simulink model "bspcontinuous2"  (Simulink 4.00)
settings: Solver=ode45  StartTime=0.0  StopTime=25  FixedStep=0.01  RelTol=1e-3
libraries: simulink3 x1

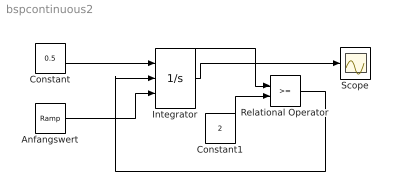
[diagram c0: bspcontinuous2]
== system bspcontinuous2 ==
  Anfangswert : simulink3/Sources/Ramp  slope=0.1  start=0  X0=0
  Constant : Constant  Value=0.5
  Constant1 : Constant  Value=2
  Integrator : Integrator  ExternalReset=rising  InitialConditionSource=external  InitialCondition=0  LimitOutput=on  UpperSaturationLimit=2  LowerSaturationLimit=-inf  ShowSaturationPort=off  ShowStatePort=on  AbsoluteTolerance=auto
  Relational Operator : RelationalOperator  Operator=>=
  Scope : Scope
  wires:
  Constant/1 -> Integrator/1
  Constant1/1 -> Relational Operator/2
  Anfangswert/1 -> Integrator/3
  Relational Operator/1 -> Integrator/2
  Integrator/1 -> Scope/1
  Integrator/State -> Relational Operator/1
